PROGRAM MAIN

VAR CONSTANT	
    cInitSource		: ST_MA_MultiArray_InitPars 
						:= ( eTypeCode := eMA_TypeCode_LREAL, nDims := 1, aDimSizes := [cBufferLength]);
END_VAR

VAR
	(* Input *)
	nInputSelection		: UDINT := 1;						// Switch between hardware and function generator	
	nSample				: UDINT;
	aEl3632 AT %I*		: ARRAY[1..cOversamples] OF INT;	// Input from hardware e.g. EL3632
	aBuffer				: ARRAY[1..cOversamples] OF LREAL;	

	// optionaly greate syntetic signal
	fbFunctionGenerator	: FB_FunctionGenerator;		// Signal Generator
	fSetFrequency		: LREAL := 50;				// Hz
	fSetAmplitude		: LREAL := 25;				// peak amplitude of sin signal		
	bAddDisturbance: BOOL := TRUE;					// add noise to sine signal if true
	fbRand: DRAND;                          
	fRandomNumber: LREAL;
	fVar: LREAL := 15;								// variance of added noise
	
	// source buffer 			
	fbSource			: FB_CMA_Source :=(	stInitPars := cInitSource, 
											nOwnID := eID_Source, 
											aDestIDs := [eID_Spectrum]);

	// sink buffers											
	fbSink				: FB_CMA_Sink := (nOwnID := eID_Sink);			// non-averaged magn. spectrum
	fbSinkAverage		: FB_CMA_Sink := (nOwnID := eID_SinkMC);		// averaged magn. spectrum
	fbSinkClassify		: FB_CMA_Sink := (nOwnID := eID_SinkClassify);	// result of classification

	aSpectrumResult			: ARRAY[1..cFFTResult] OF LREAL;
	aAverageSpectrumResult  : ARRAY[1..cFFTResult] OF LREAL; 
	aStartIdx 				: ARRAY[1..2] OF UDINT := [0,1]; 			// used for copying averaged spectrum only
	aClassificationResult	: ARRAY[1..cFFTResult] OF DINT;
	
	nCountResults			: ULINT;	
	bCalculate				: BOOL;
	bCalculateAverage		: BOOL;
	bCalculateClassifier	: BOOL;
	
	fbErrHist	: FB_HRErrHist; // error monitoring
	

	
	
END_VAR

// get input signal (I/O or signal generator)				
MAIN.InputSignal();

// call source buffer
MAIN.SourceBuffer();

// call sink buffers for (1) non-avergaged spectrum, (2) averaged spectrum, (3) classification 
MAIN.SinkBuffers();

ACTION InputSignal:

// choose between real input and function generator with added noise
CASE nInputSelection OF
	0:  (* input from EL3632 *)
		FOR nSample := 1 TO cOversamples DO
			aBuffer[nSample] := INT_TO_LREAL(aEl3632[nSample]);
		END_FOR
	1:  (* signal generator *)		
		fbFunctionGenerator(	fFrequency 	:= fSetFrequency,
								fAmplitude 	:= fSetAmplitude,
								eFunction 	:= E_FunctionType.Sine,
								aSignal		:= aBuffer );
								
		IF bAddDisturbance THEN
			// Input signal with disturbance
			FOR nSample := 1 TO cOversamples DO	
				// Random number generator	
				fbRand(Seed := 	1000, Num => fRandomNumber);			
				aBuffer[nSample] := aBuffer[nSample] + fVar*fRandomNumber;
			END_FOR
		END_IF
END_CASE
END_ACTION

ACTION SinkBuffers:

// 3 Sink buffers: (1) non-avergaged spectrum, (2) averaged spectrum, (3) classification

// (1) non-avergaged spectrum
fbSink.Output1D(	pDataOut 		:= ADR(aSpectrumResult), 
					nDataOutSize 	:= SIZEOF(aSpectrumResult), 
					eElementType 	:= eMA_TypeCode_LREAL, 
					nWorkDim 		:= 0,
					nElements		:= 0,
					pStartIndex 	:= 0,
					nOptionPars		:= 0,
					bNewResult		=> bCalculate );
IF fbSink.bError THEN
	fbErrHist.AddError(bErr:=TRUE, hrErrCode:=fbSink.hrErrorCode, sErrSource:='MAIN.fbSink'); // error monitoring
	// ToDo: if error
END_IF


// (2) averaged spectrum
fbSinkAverage.Output1D(	pDataOut 		:= ADR(aAverageSpectrumResult), 
						nDataOutSize 	:= SIZEOF(aAverageSpectrumResult), 
						eElementType 	:= eMA_TypeCode_LREAL, 
						nWorkDim 		:= 0,
						nElements		:= 0,
						pStartIndex 	:= ADR(aStartIdx),	// result of moment coeff is 2D array. Copy all frequency-bins but only second column. 
						nOptionPars		:= 0,
						bNewResult		=> bCalculateAverage );
IF fbSinkAverage.bError THEN
	fbErrHist.AddError(bErr:=TRUE, hrErrCode:=fbSinkAverage.hrErrorCode, sErrSource:='MAIN.fbSinkAverage'); // error monitoring
	// ToDo: if error
END_IF

// (3) classification
fbSinkClassify.Output1D(pDataOut 		:= ADR(aClassificationResult),
						nDataOutSize 	:= SIZEOF(aClassificationResult),
						eElementType 	:= eMA_TypeCode_INT32,
						nWorkDim 		:= 0,
						nElements 		:= 0,
						pStartIndex 	:= 0,
						nOptionPars		:= 0,
						bNewResult		=> bCalculateClassifier );						

IF fbSinkClassify.bError THEN	
	fbErrHist.AddError(bErr:=TRUE, hrErrCode:=fbSinkClassify.hrErrorCode, sErrSource:='MAIN.fbSinkClassify'); // error monitoring
END_IF
END_ACTION

ACTION SourceBuffer:


// Call source to collect data
fbSource.Input1D( pDataIn 			:= ADR(aBuffer),
				  nDataInSize 		:= SIZEOF(aBuffer), 
				  eElementType 		:= eMA_TypeCode_LREAL,
				  nWorkDim 			:= 0,
				  pStartIndex		:= 0,
				  nOptionPars		:= cCMA_Option_MarkInterruption ); 
IF fbSource.bError THEN
	fbErrHist.AddError(bErr:=TRUE, hrErrCode:=fbSource.hrErrorCode, sErrSource:='MAIN.fbSource'); // error monitoring
	// ToDo: if error
END_IF
END_ACTION

END_PROGRAM
